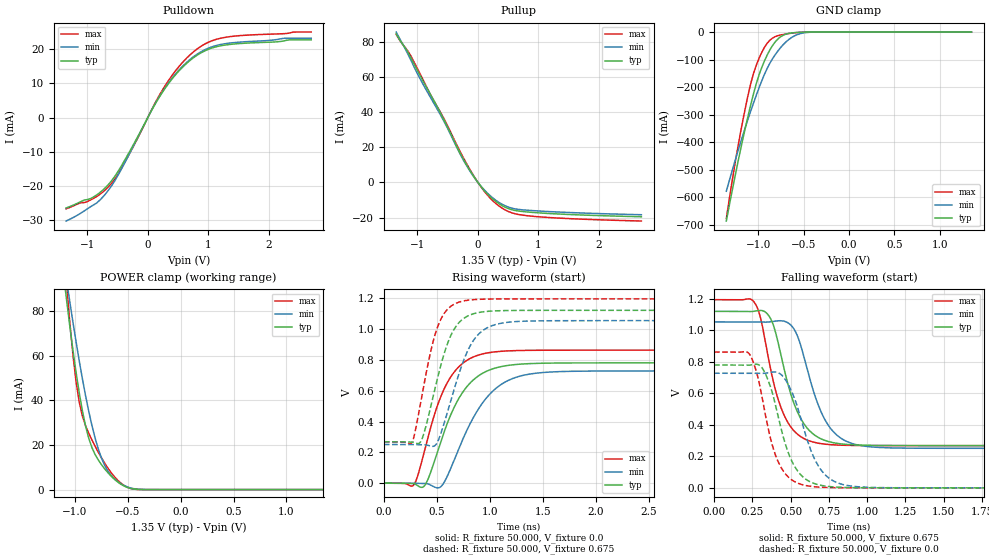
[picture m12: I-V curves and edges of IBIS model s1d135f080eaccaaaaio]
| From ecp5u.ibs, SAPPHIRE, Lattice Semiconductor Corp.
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|   Model s1d135f080eaccaaaaio
| Clamp models does not include dynamic input termination. Please
| use correspodent single-ended INPUT models to simulate input termination.
[Model] s1d135f080eaccaaaaio
Model_type I/O
Polarity   Non-Inverting
Enable   Active-Low
Vinl =  0.575V
Vinh =  0.775V
Vmeas =  0.675V
Cref =  30.000pF
Rref =  50.000
Vref =  0.675V
C_comp   5.000pF   4.000pF   5.500pF
[Temperature Range]   25.000   0.125k   -40.000
[Voltage Range]   1.350V   1.280V   1.420V
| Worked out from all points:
|   slope of the pulldown table from 0 to 0.203 V, typ, clamps not added: 31.9 ohm
|   slope of the pullup table from 0 to 0.203 V, typ, clamps not added: 25 ohm
|   GND clamp passes 1 mA (typ) near -0.54 V on its own axis
|   POWER clamp passes 1 mA (typ) near -0.51 V on its own axis
|   rising waveform, R_fixture 50.000, V_fixture 0.0: 20-80 % time 298ps typ, 346ps min, 263ps max; typ from 0 V to 0.78 V
|   rising waveform, R_fixture 50.000, V_fixture 0.675: 20-80 % time 204ps typ, 238ps min, 176ps max; typ from 0.268 V to 1.12 V
|   falling waveform, R_fixture 50.000, V_fixture 0.675: 20-80 % time 155ps typ, 167ps min, 142ps max; typ from 1.12 V to 0.268 V
|   falling waveform, R_fixture 50.000, V_fixture 0.0: 20-80 % time 141ps typ, 158ps min, 126ps max; typ from 0.78 V to 0 V
[Pulldown]
|Voltage   I(typ)   I(min)   I(max)
-1.35V    -26.53mA   -30.36mA   -26.81mA
-850mV    -22.78mA   -25.14mA   -23.23mA
-600mV    -18.58mA   -20.07mA   -19.34mA
-350mV    -11.53mA   -12.21mA   -12.18mA
50mV      1.697mA    1.729mA    1.836mA
200mV     6.283mA    6.399mA    6.82mA
450mV     12.4mA     12.61mA    13.53mA
750mV     17.5mA     17.78mA    19.22mA
1V        20.02mA    20.36mA    22.09mA
1.3V      21.34mA    21.73mA    23.6mA
2.25V     22.49mA    23.26mA    24.62mA
2.7V      22.81mA    23.26mA    25.1mA
[Pullup]
|Voltage   I(typ)   I(min)   I(max)
-1.35V    84.54mA    85.6mA     84.2mA
-1.1V     70.51mA    69.04mA    71.6mA
-800mV    51.07mA    49.36mA    51mA
-600mV    38.33mA    37.29mA    38.78mA
-200mV    10.78mA    10.31mA    11.47mA
-100mV    5.067mA    4.773mA    5.489mA
50mV      -2.275mA   -2.112mA   -2.515mA
150mV     -6.276mA   -5.848mA   -6.932mA
300mV     -10.95mA   -10.26mA   -12.1mA
550mV     -15.42mA   -14.55mA   -17.18mA
800mV     -16.76mA   -15.77mA   -18.88mA
2.7V      -19.53mA   -18.37mA   -21.95mA
[GND_clamp]
|Voltage   I(typ)   I(min)   I(max)
-1.35V    -687.3mA   -578.9mA   -678.1mA
-1.26V    -534.3mA   -475.1mA   -489.7mA
-1.2V     -438.1mA   -409.1mA   -376.7mA
-1.08V    -262.9mA   -286.2mA   -185.9mA
-1.02V    -187.7mA   -229.9mA   -120.7mA
-960mV    -129.1mA   -177.6mA   -73.95mA
-900mV    -83.6mA    -132.1mA   -40.76mA
-840mV    -48.57mA   -96.56mA   -21.66mA
-750mV    -16.65mA   -55.68mA   -10.64mA
-660mV    -4.958mA   -26.68mA   -5.448mA
-480mV    -317.7uA   -2.229mA   -341.9uA
1.35V     0A         0A         0A
[POWER_clamp]
|Voltage   I(typ)   I(min)   I(max)
-1.35V    211.5mA    193mA      324.9mA
-1.08V    85.33mA    94.25mA    92.93mA
-1.05V    73.76mA    84.65mA    75.65mA
-990mV    52.73mA    66.45mA    48.6mA
-960mV    43.53mA    57.9mA     39.38mA
-930mV    35.42mA    49.79mA    33mA
-840mV    18.88mA    28.82mA    22.31mA
-750mV    11.24mA    14.22mA    14.3mA
-660mV    6.13mA     6.499mA    7.742mA
-570mV    2.538mA    2.795mA    3.049mA
-390mV    57.41uA    134.8uA    35.81uA
1.35V     0A         0A         0A
[Ramp]
| variable   typ   min   max
dV/dt_r 0.468/0.299n   0.437/0.347n   0.518/0.264n
dV/dt_f 0.454/0.181n   0.438/0.195n   0.496/0.176n
R_load = 50.000
[Rising Waveform]
R_fixture= 50.000
V_fixture= 0.0
V_fixture_min= 0.0
V_fixture_max= 0.0
|time   V(typ)   V(min)   V(max)
0s        0V         0V         0V
284ps     -3.208mV   -430.1uV   -8.823mV
392ps     -7.27mV    -2.281mV   235.2mV
534ps     265.5mV    -24.34mV   557.6mV
637ps     454.4mV    107.5mV    696.5mV
755ps     601.6mV    302.4mV    784mV
1.027ns   742mV      597.3mV    850.3mV
1.291ns   772.5mV    695.8mV    860.9mV
1.752ns   779.9mV    725.5mV    862.9mV
10ns      780.5mV    728.2mV    862.9mV
[Rising Waveform]
R_fixture= 50.000
V_fixture= 0.675
V_fixture_min= 0.642
V_fixture_max= 0.710
|time   V(typ)   V(min)   V(max)
0s        268.3mV    251mV      268.1mV
266ps     266.4mV    250.8mV    266.4mV
358ps     284.7mV    249.7mV    567.2mV
434ps     474.8mV    241.6mV    832.9mV
493ps     646.7mV    252.2mV    988mV
632ps     960mV      539.6mV    1.148V
792ps     1.085V     861.9mV    1.187V
982ps     1.115V     1.011V     1.194V
1.352ns   1.121V     1.052V     1.196V
10ns      1.121V     1.054V     1.196V
[Falling Waveform]
R_fixture= 50.000
V_fixture= 0.675
V_fixture_min= 0.642
V_fixture_max= 0.710
|time   V(typ)   V(min)   V(max)
0s        1.121V     1.054V     1.196V
269ps     1.123V     1.055V     1.17V
308ps     1.127V     1.054V     1.062V
380ps     1.053V     1.056V     706.1mV
499ps     603.2mV    1.037V     390mV
601ps     388.1mV    782.2mV    306.6mV
736ps     297.5mV    413.5mV    276.4mV
881ps     274.8mV    289mV      269.8mV
1.177ns   268.7mV    253.3mV    268.2mV
10ns      268.3mV    251mV      268.1mV
[Falling Waveform]
R_fixture= 50.000
V_fixture= 0.0
V_fixture_min= 0.0
V_fixture_max= 0.0
|time   V(typ)   V(min)   V(max)
0s        780.5mV    728.2mV    862.9mV
234ps     780mV      728.2mV    846.1mV
288ps     783.3mV    727.8mV    696.4mV
336ps     723.8mV    728.3mV    460.3mV
442ps     360.5mV    716.4mV    122.6mV
532ps     127.1mV    551.4mV    36.6mV
657ps     26.73mV    182.9mV    6.827mV
792ps     5.096mV    37.92mV    1.168mV
1.061ns   254uV      1.992mV    48.5uV
10ns      0V         0V         0V
